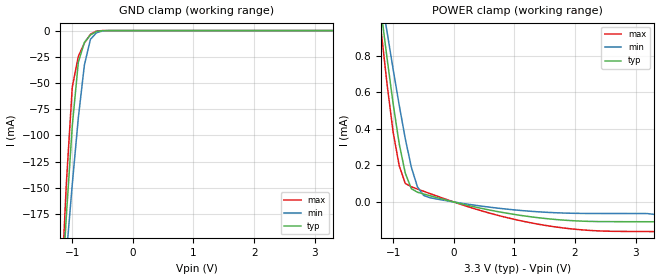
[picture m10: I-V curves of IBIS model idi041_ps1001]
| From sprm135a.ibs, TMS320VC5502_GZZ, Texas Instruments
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[Model]   idi041_ps1001
| Input with pullup
Model_type   Input
Polarity   Non-Inverting
| signals   A, Y
Vinl = 0.8V
Vinh = 2.0V
|   typ   min   max
C_comp   1.7165p   1.6246p   1.9241p
|   typ   min   max
[Temperature Range]   25   -40   125
|   typ   min   max
[Voltage Range]   3.30V   3.00V   3.60V
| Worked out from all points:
|   GND clamp passes 1 mA (typ) near -0.61 V on its own axis
|   POWER clamp passes 1 mA (typ) near -1.18 V on its own axis
[GND_clamp]
|   Voltage   I(typ)   I(min)   I(max)
-3.3V     -2.557A    -1.931A    -3.318A
-1.2V     -276.8mA   -288.6mA   -274mA
-1.1V     -179.1mA   -216.2mA   -148.3mA
-1V       -90.91mA   -146.8mA   -53.98mA
-900mV    -30.19mA   -83.19mA   -24.6mA
-800mV    -11.29mA   -32.84mA   -11.96mA
-700mV    -4.166mA   -8.321mA   -3.542mA
-600mV    -817.5uA   -2.039mA   -409.4uA
-500mV    -75.2uA    -367.8uA   -19.35uA
-400mV    -4.217uA   -45.04uA   -434.7nA
3.3V      222pA      35.04nA    133.2pA
[POWER_clamp]
|   Voltage   I(typ)   I(min)   I(max)
-3.3V     6.905mA    5.744mA    7.841mA
-1.2V     1.047mA    1.139mA    943.6uA
-1.1V     786.2uA    930.8uA    644.3uA
-1V       537.8uA    726.9uA    382uA
-900mV    318.6uA    530.3uA    198.8uA
-800mV    158.1uA    346.8uA    101.7uA
-700mV    72.97uA    190.9uA    83uA
-600mV    53.62uA    83.38uA    70.93uA
-500mV    44.09uA    36.26uA    58.94uA
500mV     -38.02uA   -24.54uA   -52.48uA
1.4V      -86.42uA   -53.96uA   -122uA
3.3V      -108.3uA   -67.64uA   -162.1uA
